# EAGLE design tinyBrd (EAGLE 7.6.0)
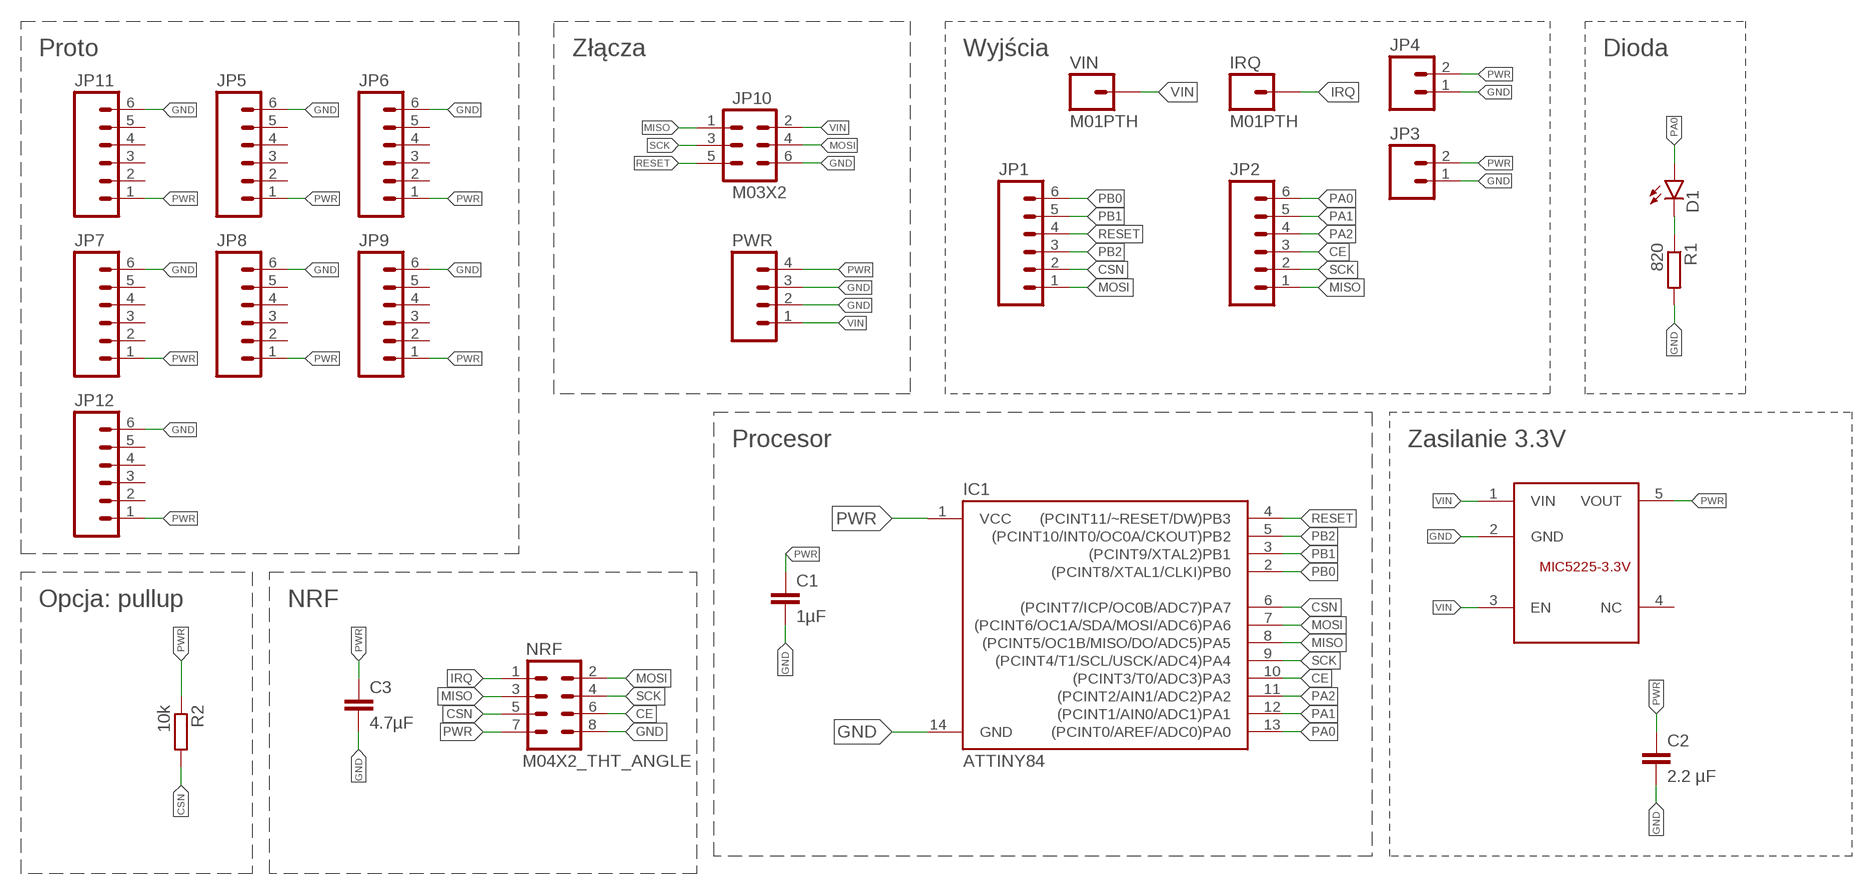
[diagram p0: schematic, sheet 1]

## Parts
C1  1µF  C-EUC0805  [C0805]
C2  2.2 µF  C-EUC0805  [C0805]
C3  4.7µF  C-EUC0805  [C0805]
D1  LED0603  [LED-0603]
IC1  ATTINY84  [SO14]
IC2  MIC5225  [SOT23-5L]
IRQ  M01PTH  [1X01]
JP1  M06SILK_FEMALE_PTH  [1X06]
JP2  M06SILK_FEMALE_PTH  [1X06]
JP3  M02PTH  [1X02]
JP4  M02PTH  [1X02]
JP5  M06SILK_FEMALE_PTH  [1X06]
JP6  M06SILK_FEMALE_PTH  [1X06]
JP7  M06SILK_FEMALE_PTH  [1X06]
JP8  M06SILK_FEMALE_PTH  [1X06]
JP9  M06SILK_FEMALE_PTH  [1X06]
JP10  M03X2  [2X3-SMD]
JP11  M06SILK_FEMALE_PTH  [1X06]
JP12  M06SILK_FEMALE_PTH  [1X06]
NRF  M04X2_THT_ANGLE  2X4SMD_ANG  [2X4_SMD_ANGLE]
PWR  M04PTH  [1X04]
R1  820  R-EU_R0805  [R0805]
R2  10k  R-EU_R0603  [R0603]
VIN  M01PTH  [1X01]

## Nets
CE: IC1.10((PCINT3/T0/ADC3)PA3) JP2.3 NRF.6
CSN: IC1.6((PCINT7/ICP/OC0B/ADC7)PA7) JP1.2 NRF.5 R2.2
GND: C1.2 C2.2 C3.2 IC1.14(GND) IC2.2(GND) JP3.1 JP4.1 JP5.6 JP6.6 JP7.6 JP8.6 JP9.6 JP10.6 JP11.6 JP12.6 NRF.8 PWR.2 PWR.3 R1.2
IRQ: IRQ.1 NRF.1
MISO: IC1.8((PCINT5/OC1B/MISO/DO/ADC5)PA5) JP2.1 JP10.1 NRF.3
MOSI: IC1.7((PCINT6/OC1A/SDA/MOSI/ADC6)PA6) JP1.1 JP10.4 NRF.2
N$5: D1.C R1.1
PA0: D1.A IC1.13((PCINT0/AREF/ADC0)PA0) JP2.6
PA1: IC1.12((PCINT1/AIN0/ADC1)PA1) JP2.5
PA2: IC1.11((PCINT2/AIN1/ADC2)PA2) JP2.4
PB0: IC1.2((PCINT8/XTAL1/CLKI)PB0) JP1.6
PB1: IC1.3((PCINT9/XTAL2)PB1) JP1.5
PB2: IC1.5((PCINT10/INT0/OC0A/CKOUT)PB2) JP1.3
PWR: C1.1 C2.1 C3.1 IC1.1(VCC) IC2.5(VOUT) JP3.2 JP4.2 JP5.1 JP6.1 JP7.1 JP8.1 JP9.1 JP11.1 JP12.1 NRF.7 PWR.4 R2.1
RESET: IC1.4((PCINT11/~RESET/DW)PB3) JP1.4 JP10.5
SCK: IC1.9((PCINT4/T1/SCL/USCK/ADC4)PA4) JP2.2 JP10.3 NRF.4
VIN: IC2.1(VIN) IC2.3(EN) JP10.2 PWR.1 VIN.1
Unconnected: IC2.4(NC) JP5.2 JP5.3 JP5.4 JP5.5 JP6.2 JP6.3 JP6.4 JP6.5 JP7.2 JP7.3 JP7.4 JP7.5 JP8.2 JP8.3 JP8.4 JP8.5 JP9.2 JP9.3 JP9.4 JP9.5 JP11.2 JP11.3 JP11.4 JP11.5 JP12.2 JP12.3 JP12.4 JP12.5

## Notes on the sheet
- Proto | Złącza | Wyjścia | Dioda
- Procesor | Zasilanie 3.3V
- Opcja: pullup | NRF

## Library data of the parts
C1 C3 = rcl:C-EU: CAPACITOR, European symbol
C2 = resistor:C-EU: CAPACITOR, European symbol
D1 = nettigo:LED: LEDs
IC1 = SparkFun-DigitalIC:ATTINY84: Atmel 14-pin 2/4/8kB flash uC; PROD_ID: IC-11285
IC2 = nettigo:MIC5225
IRQ VIN = SparkFun-Connectors:M01: Header 1
JP1 JP2 JP5-JP9 JP11 JP12 = SparkFun-Connectors:M06: Header 6 Standard 6-pin 0.1" header. Use with straight break away headers (SKU : PRT-00116), right angle break away headers (PRT-00553), swiss pins (PRT-00743), machine pins (PRT-00117), and female headers (PRT-00115). Molex polarized connector foot print use with SKU : PRT-08094 with associated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; PROD_ID: CONN-08437
JP3 JP4 = SparkFun-Connectors:M02: Standard 2-pin 0.1" header. Use with
JP10 = nettigo:M03X2
NRF = nettigo:2X4: .1" header, two rows of four.
PWR = SparkFun-Connectors:M04: Header 4 Standard 4-pin 0.1" header. Use with straight break away headers (SKU : PRT-00116), right angle break away headers (PRT-00553), swiss pins (PRT-00743), machine pins (PRT-00117), and female headers (PRT-00115). Molex polarized connector foot print use with SKU : PRT-08231 with associated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
R1 R2 = rcl:R-EU_: RESISTOR, European symbol

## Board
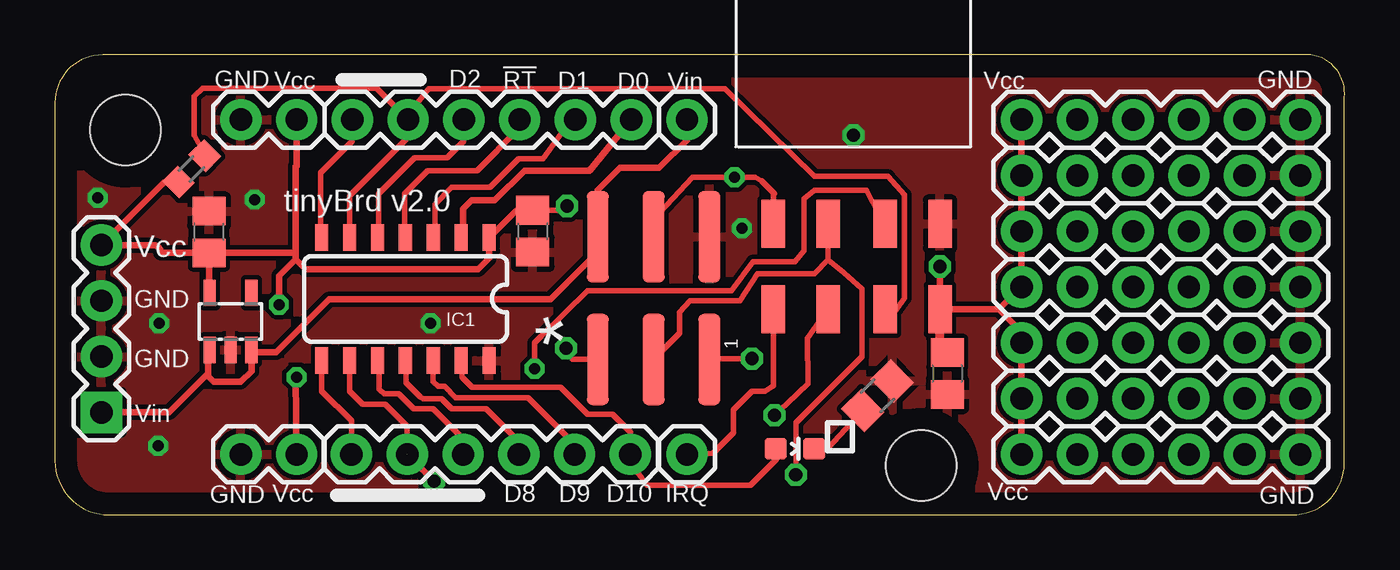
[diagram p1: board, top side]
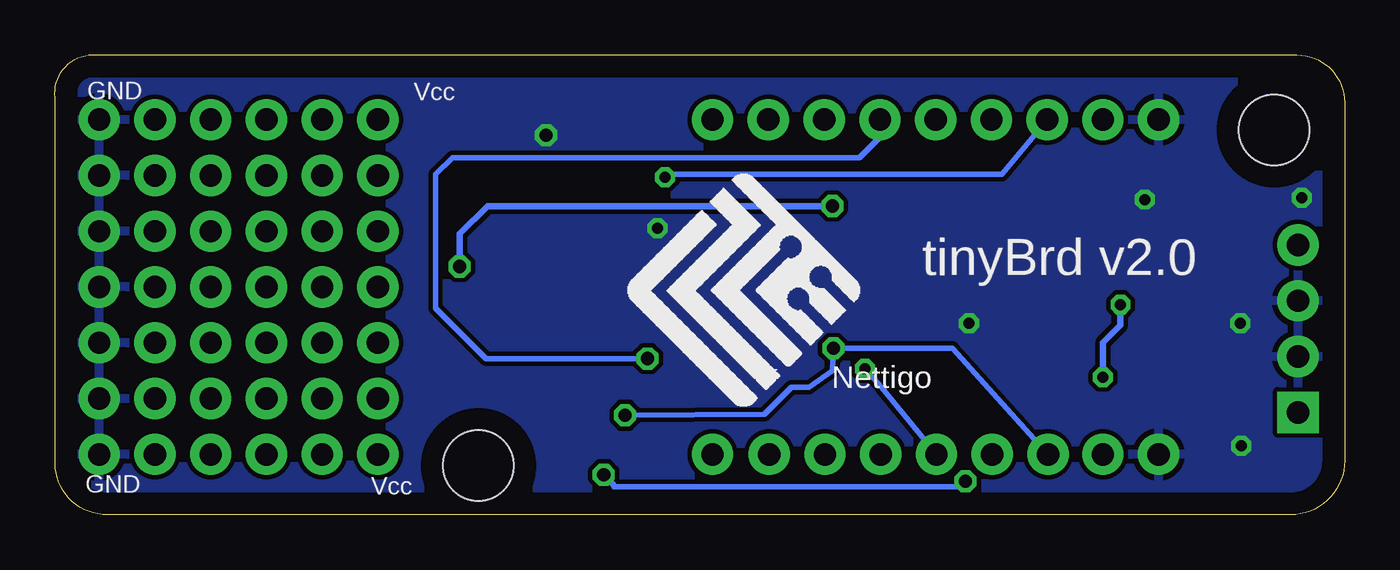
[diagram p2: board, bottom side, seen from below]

Size 58.74 x 20.94 mm. Coordinates in mm from the lower left corner, seen from the top.
Outline: 2.46,0 56.36,0 arc90 58.73,2.34 58.73,18.99 arc90 57.2,20.94 2.17,20.94 arc90 0,18.76 0,2.46 arc90 2.46,0
Copper layers (1*16): Top 0.035mm / dielectric 1.5mm / Bottom 0.035mm
Design rules "default": minimum track width 10mil, minimum drill 24mil, track to track 8mil, track to pad 8mil, pad to pad 8mil, via to via 8mil, smd to smd 8mil, copper to edge 40mil, drill to drill 8mil, minimum pad ring 10mil, minimum via ring 8mil, stop-mask expansion 4mil, vias tented up to drill 0mil, thermal gap 10mil
Holes 3.2 mm at 3.21,17.53 39.46,2.24

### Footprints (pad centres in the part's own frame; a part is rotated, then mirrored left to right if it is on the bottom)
C0805 = smd 1.3 x 1.5: 1 -0.95,0; 2 0.95,0
LED-0603 = smd 1 x 1: A 0,-0.877; C 0,0.877
SO14 = smd 0.6 x 1.2: 1 -3.81,-2.8; 2 -2.54,-2.8; 3 -1.27,-2.8; 4 0,-2.8; 5 1.27,-2.8; 6 2.54,-2.8; 7 3.81,-2.8; 8 3.81,2.8; 9 2.54,2.8; 10 1.27,2.8; 11 0,2.8; 12 -1.27,2.8; 13 -2.54,2.8; 14 -3.81,2.8
SOT23-5L = smd 0.55 x 1.2: 1 -0.95,-1.3; 2 0,-1.3; 3 0.95,-1.3; 4 0.95,1.3; 5 -0.95,1.3
1X01 = drill 1.016 pad 1.88: 1 0,0
1X06 = drill 1.016 pad 1.88: 1 0,0; 2 2.54,0; 3 5.08,0; 4 7.62,0; 5 10.16,0; 6 12.7,0
1X02 = drill 1.016 pad 1.88: 1 0,0; 2 2.54,0
2X3-SMD = smd 4.15 x 1: 1 -2.794,2.54; 2 2.794,2.54; 3 -2.794,0; 4 2.794,0; 5 -2.794,-2.54; 6 2.794,-2.54
2X4_SMD_ANGLE = smd 2.184 x 1.067: 1 -2,3.7; 2 1.9,3.7; 3 -2,1.2; 4 1.9,1.2; 5 -2,-1.4; 6 1.9,-1.4; 7 -2,-3.9; 8 1.9,-3.9
1X04 = drill 1.016 pad 1.88 square: 1 0,0 | drill 1.016 pad 1.88: 2 2.54,0; 3 5.08,0; 4 7.62,0
R0805 = smd 1.3 x 1.5: 1 -0.95,0; 2 0.95,0
R0603 = smd 1 x 1.1: 1 -0.85,0; 2 0.85,0

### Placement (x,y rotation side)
C1  21.76,12.91 270 top
C2  7.02,12.87 90 top
C3  40.65,6.44 270 top
D1  33.7,3.01 270 top
IC1  15.97,9.82 180 top
IC2  8,8.81 0 top
IRQ  28.79,2.75 0 top
JP1  13.55,17.99 0 top
JP2  13.51,2.75 0 top
JP3  8.47,2.75 0 top
JP4  8.47,17.99 0 top
JP5  44.03,17.99 0 top
JP6  44.03,15.45 0 top
JP7  44.03,10.37 0 top
JP8  44.03,7.83 0 top
JP9  44.03,5.29 0 top
JP10  27.27,9.87 90 top
JP11  44.03,2.75 0 top
JP12  44.03,12.91 0 top
NRF  36.42,11.35 90 top
PWR  2.12,4.66 90 top
R1  37.47,5.42 45 top
R2  6.22,15.75 45 top
VIN  28.79,17.99 0 top

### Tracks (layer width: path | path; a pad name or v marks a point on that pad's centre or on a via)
CE  (via drill 0.5 pad 0.25)
  Top 0.254: IC1.10 14.78,6.94 14.78,5.72 14.99,5.5 15.67,5.5 16.34,4.83 17.23,4.83 18.59,3.47 JP2.3 | NRF.6 37.82,13.12 36.96,14.78 34.59,14.78 34.13,14.4 34.13,12.03 33.7,11.52 31.8,11.52 30.82,10.2 24.26,10.2 22.14,8.13 21.85,7.83 v21.85,6.65
  Bottom 0.254: v21.85,6.65 21.09,5.8 JP2.3
CSN
  Top 0.254: IC1.6 13.42,14.52 16.09,17.19 | 16.09,17.19 JP1.2 14.65,19.43 6.73,19.43 6.35,19.05 6.35,17.27 6.67,16.7 R2.2 | 16.09,17.19 16.09,18.21 17.02,19.39 30.53,19.39 34.59,15.41 37.94,15.41 38.7,14.57 38.7,9.87 37.82,8.65 NRF.5
GND  (via drill 0.5 pad 0.25, 0.5 pad 0.3, 0.6)
  other vias: 36.37,17.28 31.29,13.04 4.7,3.13 1.95,14.44 9.1,14.35 4.74,8.72 17.11,8.72
  pour Top: 0.04,19.77 61.13,19.72 61.09,-1.14 0,0
  pour Bottom: 0.21,20.15 0,-0.51 61.01,-1.44 60.33,19.72
IRQ
  Top 0.254: IRQ.1 29.98,2.79 30.91,3.73 30.91,4.79 31.76,5.63 32.35,5.63 32.72,5.88 NRF.1
MISO  (via drill 0.6)
  Top 0.254: IC1.8 12.16,5.63 13.51,4.27 JP2.1 | JP10.1 23.58,7.07 v23.29,7.58 | NRF.3 34.29,8.04 34.3,5.97 33.37,5.08 v32.77,4.53
  Bottom 0.254: JP2.1 17.86,7.58 v23.29,7.58 23.33,6.56 24.39,5.8 25.19,5.8 26.42,4.57 v32.77,4.53
MOSI  (via drill 0.5 pad 0.25)
  Top 0.254: IC1.7 12.11,12.67 12.11,15.58 13.55,17.02 JP1.1 | JP10.4 27.27,13.46 29.05,15.37 v30.95,15.37 31.88,15.37 32.18,15.2 | 32.18,15.2 | 32.18,15.2 32.77,14.61 32.72,14.61 NRF.2
  Bottom 0.254: v30.95,15.37 30.83,15.49 29.34,15.49 15.61,15.5 JP1.1
N$5
  Top 0.254: D1.C 35.19,3.01 R1.1
PA0
  Top 0.254: IC1.13 18.55,6.98 18.55,6.27 19.01,5.8 23.03,5.8 24.26,4.57 25.41,4.57 26.21,3.77 JP2.6 26.21,3.27 26.21,2.37 26.97,1.35 31.68,1.35 32.86,2.53 32.86,2.58 D1.A
PA1
  Top 0.254: IC1.12 17.23,6.05 17.45,5.84 17.74,5.84 18.25,5.33 21.55,5.33 23.62,3.27 JP2.5
PA2
  Top 0.254: IC1.11 16,6.98 16,6.01 16.64,5.38 16.77,5.29 17.61,5.29 18.08,4.83 19.65,4.83 21.13,3.34 JP2.4
PB0
  Top 0.305: IC1.2 18.59,12.7 18.59,13.93 18.97,14.31 20.03,14.31 21.38,15.67 24.35,15.67 JP1.6
PB1
  Top 0.254: IC1.3 17.32,12.7 17.32,14.14 18.08,14.9 19.82,14.9 21.13,16.22 22.23,16.22 23.58,18.07 JP1.5
PB2
  Top 0.254: IC1.5 14.73,12.66 14.73,14.61 16.39,16.26 17.87,16.26 18.63,17.02 JP1.3
PWR  (via drill 0.5 pad 0.3, 0.6)
  Top 0.254: IC1.1 | v23.33,14.06 23.14,13.86 C1.1 21.02,13.86 IC1.1
  Top 0.305: JP4.2 11.01,15.88 arc90 10.97,15.84 10.97,11.94 | IC1.1 | v40.31,11.3 40.32,9.94 NRF.7 43.01,9.35 | IC1.1 19.77,11.69 19.27,11.18 11.43,11.18 10.97,11.64 | 10.97,11.64 10.97,11.94 | JP3.2 10.97,6.22 v11.01,6.27 | v10.2,9.57 10.2,10.88 10.97,11.64 | IC2.5 7.03,10.11 C2.1 7.03,11.94 | 7.03,11.94 4.83,11.94 arc90 4.48,12.28 PWR.4 4.95,15.11 R2.1 | 7.03,11.94 10.97,11.94 | 43.01,9.35 JP7.1 JP12.1 JP6.1 JP5.1 | 43.01,9.35 44.03,8.33 JP8.1 JP9.1 JP11.1
  Top 0.406: C3.1 40.32,7.39 NRF.7
  Bottom 0.305: 10.97,17.53 JP4.2 | v23.33,14.06 39.04,14.06 40.31,12.79 v40.31,11.3 40.31,11.35 40.39,11.35 40.61,11.56 | v11.01,6.27 11.01,7.83 10.2,8.64 v10.2,9.57
RESET  (via drill 0.6 pad 0.25)
  Top 0.254: IC1.4 15.92,12.67 15.92,14.61 16.98,15.67 19.22,15.67 21.12,17.57 JP1.4 | JP10.5 29.85,7.11 v31.75,7.11
  Bottom 0.254: v31.75,7.11 39.12,7.11 41.4,9.4 41.4,15.49 40.64,16.26 22.1,16.26 21.17,17.19 JP1.4
SCK  (via drill 0.6 pad 0.25)  (1 unrouted)
  Top 0.254: IC1.9 13.42,5.63 14.02,5.04 15.03,5.04 16.05,4.02 JP2.2 v17.27,1.52 | NRF.4 35.22,11.61 | 35.22,11.61 35.95,11.01 36.75,10.29 36.75,7.2 33.75,4.19 v33.75,1.82 | JP10.3 28.45,8.26 28.45,9.23 28.92,9.74 31.21,9.74 32.01,10.97 34.59,10.97 34.6,10.97 35.22,11.61
  Bottom 0.254: v17.27,1.52 17.53,1.27 33.27,1.27 33.27,1.35 v33.75,1.82
VIN
  Top 0.305: IC2.1 6.99,7.44 6.99,6.44 | 6.99,6.44 6.99,6.31 7.24,6.05 8.47,6.05 8.95,6.54 IC2.3 9.05,7.41 10.08,7.41 12.49,9.82 22.57,9.82 24.73,11.98 JP10.2 | JP10.2 | JP10.2 24.73,14.78 25.74,15.79 27.52,15.79 28.79,17.06 VIN.1 | PWR.1 5.21,4.66 6.99,6.44

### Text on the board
tNames: GND | Vcc | D2 | !RT | D1 | D0 | Vin | Vcc | GND | tinyBrd v2.0 | Vcc | GND | * | GND | Vin | GND | Vcc | D8 | D9 | D10 | IRQ | Vcc | GND
bNames: Vcc | GND | tinyBrd v2.0 | Nettigo | Vcc | GND
tDocu: v2.0 / Zmiany do v1.5 / - miejsce na pullup do CSN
